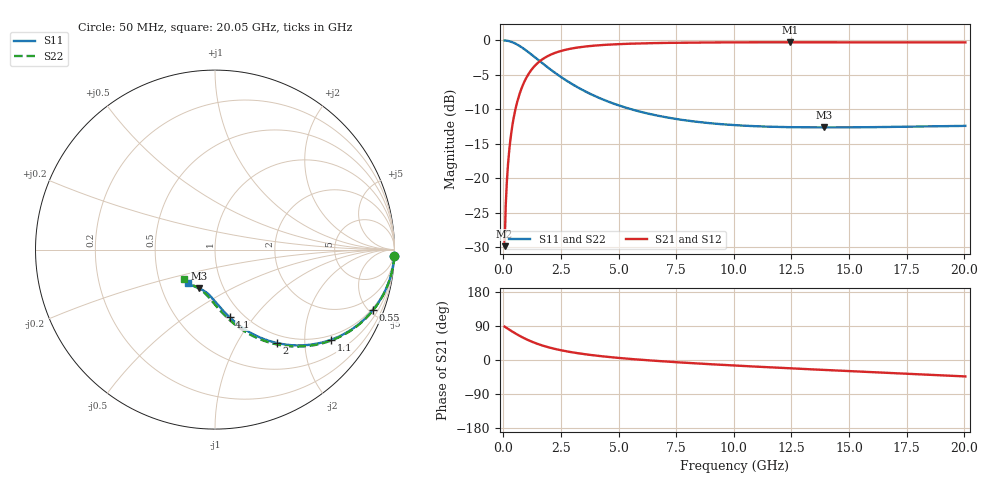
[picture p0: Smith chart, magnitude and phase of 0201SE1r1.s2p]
! AVX Thin Film Operation		Date: August 2001
! Description: Accu-P® Series, Thin Film, SMD, RF Capacitor
! Part Number: 02013J1R1ABW
! 50 MHz  -  20.05 GHz
! Serial Measurements
# mhz S db R 50
!	S11		S21		S12		S22
!	dB	Phase	dB	Phase	dB	Phase	dB	Phase
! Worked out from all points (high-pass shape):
!   401 points, 50 MHz to 20.05 GHz, reference 50 ohm
!   highest |S21| = -0.26 dB at 12.45 GHz (marker M1); lowest = -29.9 dB at 50 MHz (marker M2)
!   |S21| within 3 dB of the highest: 1.491 GHz to end of sweep
!   lowest |S11| = -12.6 dB at 13.9 GHz (marker M3), VSWR 1.61, Z = 38.4 - j17.5 ohm
!   |S11| at or under -10 dB: 5.557 GHz to end of sweep
!   |S22| runs from -12.7 to 0.0 dB; largest |S21 - S12| = 0
!   S11 on the Smith chart (normalised r, x): 50 MHz: 1, -58; 550 MHz: 0.88, -5.29; 1.1 GHz: 0.87, -2.66; 2 GHz: 0.87, -1.48; 4.1 GHz: 0.86, -0.77; 20.05 GHz: 0.70, -0.28
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50  -0.00 -2.0  -29.86 88.0  -29.86 88.0  -0.00 -2.0
100  -0.02 -3.9  -23.85 86.0  -23.85 86.0  -0.02 -4.0
200  -0.07 -7.8  -17.88 82.1  -17.88 82.1  -0.07 -8.0
250  -0.11 -9.8  -15.99 80.1  -15.99 80.1  -0.11 -9.9
300  -0.16 -11.7  -14.45 78.2  -14.45 78.2  -0.16 -11.9
400  -0.28 -15.5  -12.08 74.4  -12.08 74.4  -0.28 -15.7
550  -0.51 -20.9  -9.55 69.0  -9.55 69.0  -0.51 -21.2
800  -1.01 -29.2  -6.82 60.5  -6.82 60.5  -1.01 -29.6
1100  -1.74 -37.9  -4.82 51.7  -4.82 51.7  -1.74 -38.5
1500  -2.80 -47.4  -3.24 42.1  -3.24 42.1  -2.81 -48.2
2000  -4.11 -56.6  -2.14 32.8  -2.14 32.8  -4.11 -57.6
2650  -5.65 -65.3  -1.39 23.9  -1.39 23.9  -5.65 -66.7
3400  -7.13 -72.6  -0.95 16.4  -0.95 16.4  -7.13 -74.3
4100  -8.26 -77.8  -0.71 11.0  -0.71 11.0  -8.27 -79.9
5250  -9.69 -84.3  -0.51 4.1  -0.51 4.1  -9.70 -87.0
6750  -10.96 -90.8  -0.38 -2.8  -0.38 -2.8  -10.97 -94.2
10050  -12.29 -101.7  -0.28 -14.6  -0.28 -14.6  -12.32 -106.6
12450  -12.59 -108.5  -0.26 -22.0  -0.26 -22.0  -12.62 -114.4
13400  -12.62 -111.0  -0.26 -24.7  -0.26 -24.7  -12.66 -117.4
13900  -12.63 -112.3  -0.27 -26.2  -0.27 -26.2  -12.67 -118.9
16750  -12.55 -119.7  -0.27 -34.2  -0.27 -34.2  -12.61 -127.5
20050  -12.40 -128.1  -0.28 -43.4  -0.28 -43.4  -12.46 -137.4
